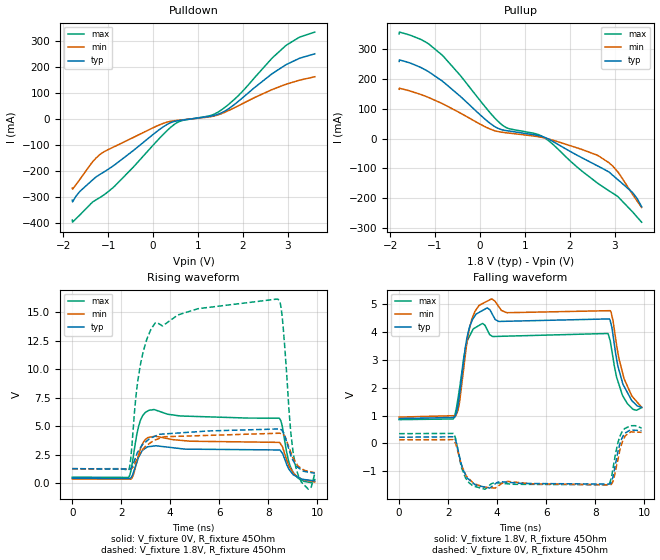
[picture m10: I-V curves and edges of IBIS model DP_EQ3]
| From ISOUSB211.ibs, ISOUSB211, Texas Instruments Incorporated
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[Model]   DP_EQ3
Model_type   Output
Polarity   Non-Inverting
Vmeas = 0.2
Vref = 0
Cref = 15pF
Rref = 45
|   typ   min   max
C_comp   5pF   3pF   8pF
[Voltage Range]   1.8   1.71   1.89
[Temperature Range]   27   150   -40
[Pullup Reference]   1.8   1.71   1.89
[Pulldown Reference]   0   0   0
[Power Clamp Reference]   1.8   1.71   1.89
[GND Clamp Reference]   0   0   0
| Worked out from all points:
|   slope of the pulldown table from 0 to 0.27 V, typ, clamps not added: 7.95 ohm
|   slope of the pullup table from 0 to 0.27 V, typ, clamps not added: 7.94 ohm
|   falling waveform, V_fixture 1.8V, R_fixture 45Ohm: 20-80 % time 84.1ps typ, 85.9ps min, 83.5ps max; typ from 0.895 V to 1.3 V
|   rising waveform, V_fixture 0V, R_fixture 45Ohm: 20-80 % time 402ps typ, 364ps min, 86.9ps max; typ from 0.46 V to 0.225 V
|   rising waveform, V_fixture 1.8V, R_fixture 45Ohm: 20-80 % time 348ps typ, 328ps min, 35.7ps max; typ from 1.3 V to 0.895 V
|   falling waveform, V_fixture 0V, R_fixture 45Ohm: 20-80 % time 155ps typ, 162ps min, 102ps max; typ from 0.225 V to 0.46 V
[Pulldown]
|   Voltage   I(typ)   I(min)   I(max)
-1.8V     -312.3mA   -266.2mA   -388.8mA
-1.795V   -319mA     -269.8mA   -396.8mA
-1.633V   -278.9mA   -232.8mA   -369.2mA
-1.179V   -212.7mA   -136mA     -301.6mA
-865.8mV  -177.8mA   -106.8mA   -260mA
73.8mV    -49.63mA   -27.98mA   -87.09mA
538.2mV   -7.266mA   -5.626mA   -13.71mA
1.294V    10.85mA    9.019mA    13.98mA
1.521V    23.18mA    20.15mA    34.45mA
1.899V    67.71mA    50.57mA    89.7mA
2.947V    206.8mA    132.3mA    280.4mA
3.6V      250.2mA    161.9mA    333.6mA
[Pullup]
|   Voltage   I(typ)   I(min)   I(max)
-1.8V     259.8mA    166.3mA    352.1mA
-1.795V   264.8mA    169.7mA    358.5mA
-1.325V   240.1mA    149.1mA    334.3mA
-849.6mV  194.9mA    118.9mA    282mA
381.6mV   36.3mA     24.84mA    61.51mA
613.8mV   26.64mA    19.55mA    35.63mA
1.402V    6.733mA    3.773mA    6.537mA
2.612V    -90.76mA   -55.24mA   -148.5mA
2.876V    -112.3mA   -81.28mA   -175.5mA
3.065V    -136.9mA   -110.7mA   -193.6mA
3.4V      -181.3mA   -187.3mA   -246.2mA
3.6V      -228.6mA   -231.2mA   -280.5mA
[Ramp]
R_load = 45
|   typ   min   max
dV/dt_r   0.140808/3.11889e-10   0.160407/2.9261e-10   0.120509/5.38843e-09
dV/dt_f   0.243789/7.74248e-11   0.210518/8.21241e-11   0.256824/7.47009e-09
[Falling Waveform]
V_fixture = 1.8V
V_fixture_min = 1.71V
V_fixture_max = 1.89V
R_fixture = 45Ohm
C_fixture = 0F
|   Time   V(typ)   V(min)   V(max)
0s        895mV      947.6mV    856.5mV
2.316ns   1.048V     999.9mV    1.184V
2.644ns   3.048V     2.762V     3.125V
2.883ns   4.207V     4.172V     3.872V
3.403ns   4.778V     5.025V     4.309V
3.757ns   4.72V      5.189V     3.874V
4.392ns   4.391V     4.698V     3.856V
8.615ns   4.417V     4.772V     3.699V
9.13ns    2.148V     2.512V     1.713V
9.9ns     1.301V     1.298V     1.285V
[Rising Waveform]
V_fixture = 0V
V_fixture_min = 0V
V_fixture_max = 0V
R_fixture = 45Ohm
C_fixture = 0F
|   Time   V(typ)   V(min)   V(max)
0s        459.5mV    400.3mV    553.4mV
2.295ns   442.5mV    378.8mV    530.3mV
2.502ns   999.3mV    791.9mV    2.512V
2.779ns   2.581V     3.002V     5.513V
3.326ns   3.279V     4.118V     6.478V
8.436ns   2.938V     3.602V     5.727V
8.565ns   2.689V     3.269V     5.098V
8.821ns   1.353V     1.682V     2.054V
9.008ns   801.9mV    980.3mV    1.009V
9.9ns     224.9mV    133mV      352.5mV
[Rising Waveform]
V_fixture = 1.8V
V_fixture_min = 1.71V
V_fixture_max = 1.89V
R_fixture = 45Ohm
C_fixture = 0F
|   Time   V(typ)   V(min)   V(max)
0s        1.301V     1.298V     1.285V
2.304ns   1.26V      1.259V     1.168V
2.766ns   3.079V     2.688V     10.24V
3.377ns   4.145V     3.808V     14.04V
8.364ns   4.774V     4.398V     16.16V
8.56ns    4.663V     4.351V     14.83V
8.913ns   2.528V     2.792V     4.689V
9.11ns    1.65V      1.892V     1.593V
9.632ns   996.3mV    1.073V     -485.9mV
9.9ns     895mV      947.6mV    856.5mV
[Falling Waveform]
|Gnd
V_fixture = 0V
V_fixture_min = 0V
V_fixture_max = 0V
R_fixture = 45Ohm
C_fixture = 0F
|   Time   V(typ)   V(min)   V(max)
0s        224.9mV    133mV      352.5mV
2.207ns   239mV      136.6mV    361.3mV
2.711ns   -1.125V    -1.114V    -1.239V
3.487ns   -1.564V    -1.57V     -1.642V
3.895ns   -1.468V    -1.6V      -1.41V
8.544ns   -1.46V     -1.485V    -1.483V
8.754ns   -1.105V    -1.302V    -781.9mV
9.093ns   177.7mV    3.11mV     407.8mV
9.461ns   484.1mV    417.9mV    636.9mV
9.9ns     459.5mV    400.3mV    553.4mV
